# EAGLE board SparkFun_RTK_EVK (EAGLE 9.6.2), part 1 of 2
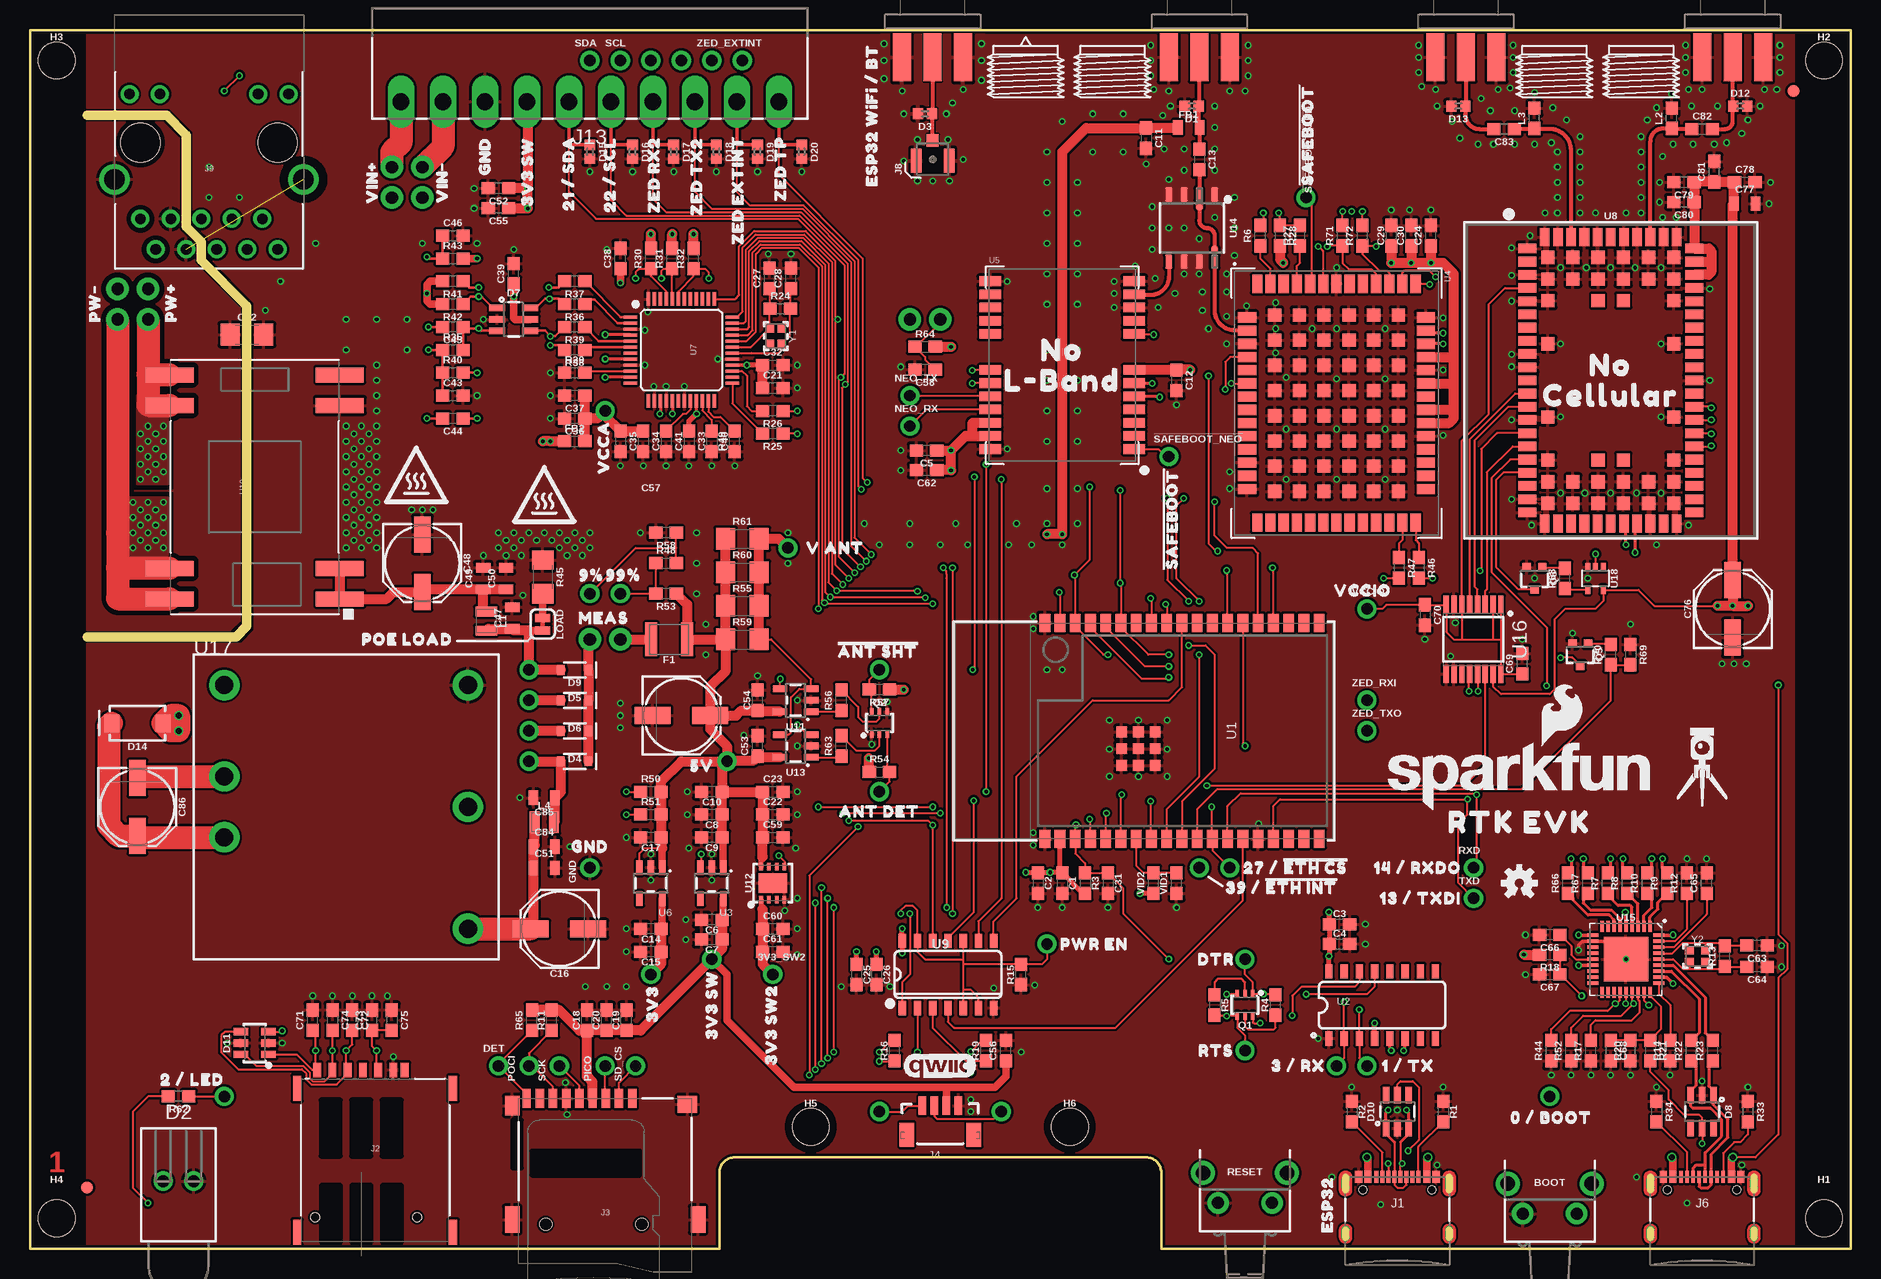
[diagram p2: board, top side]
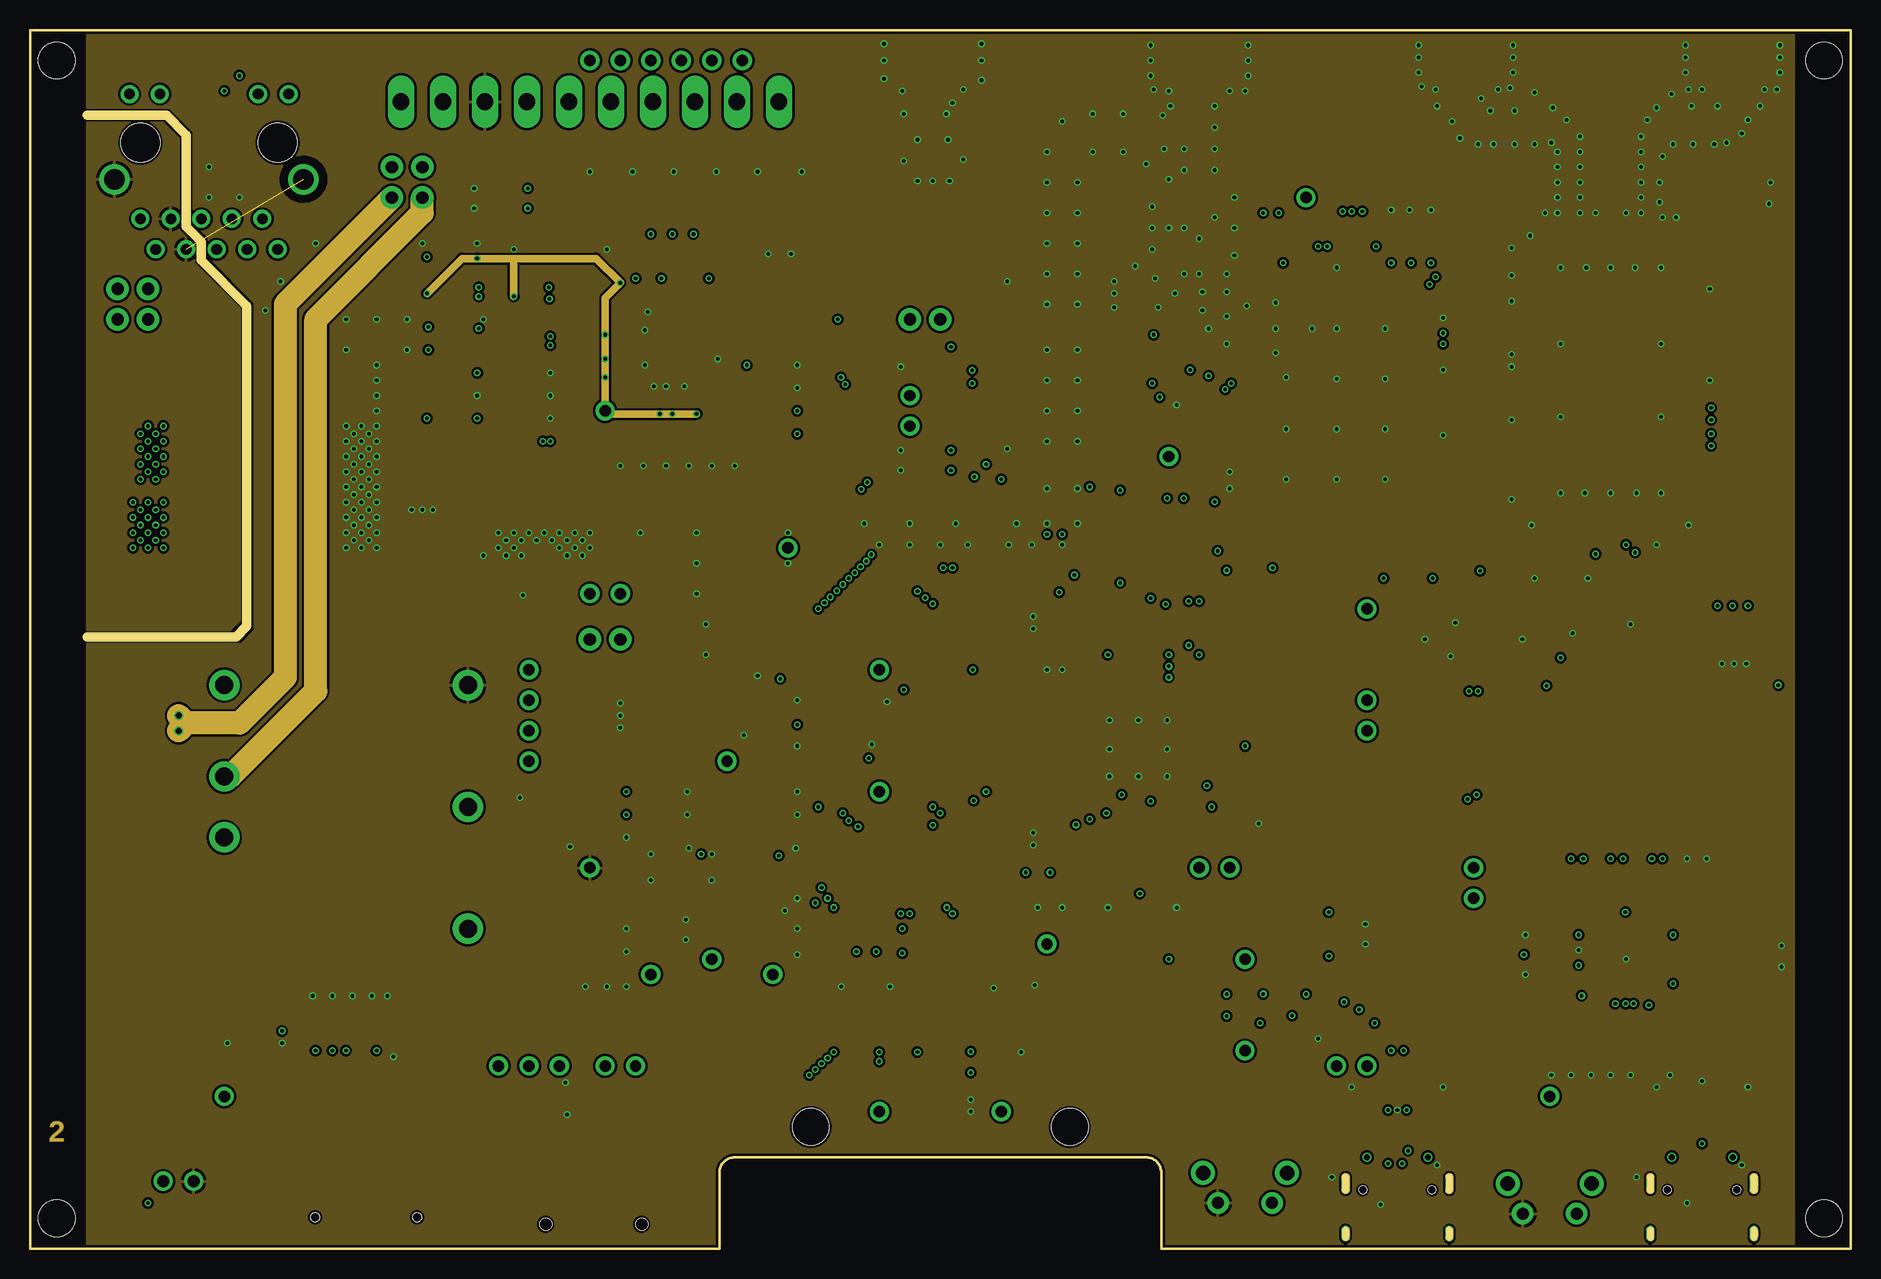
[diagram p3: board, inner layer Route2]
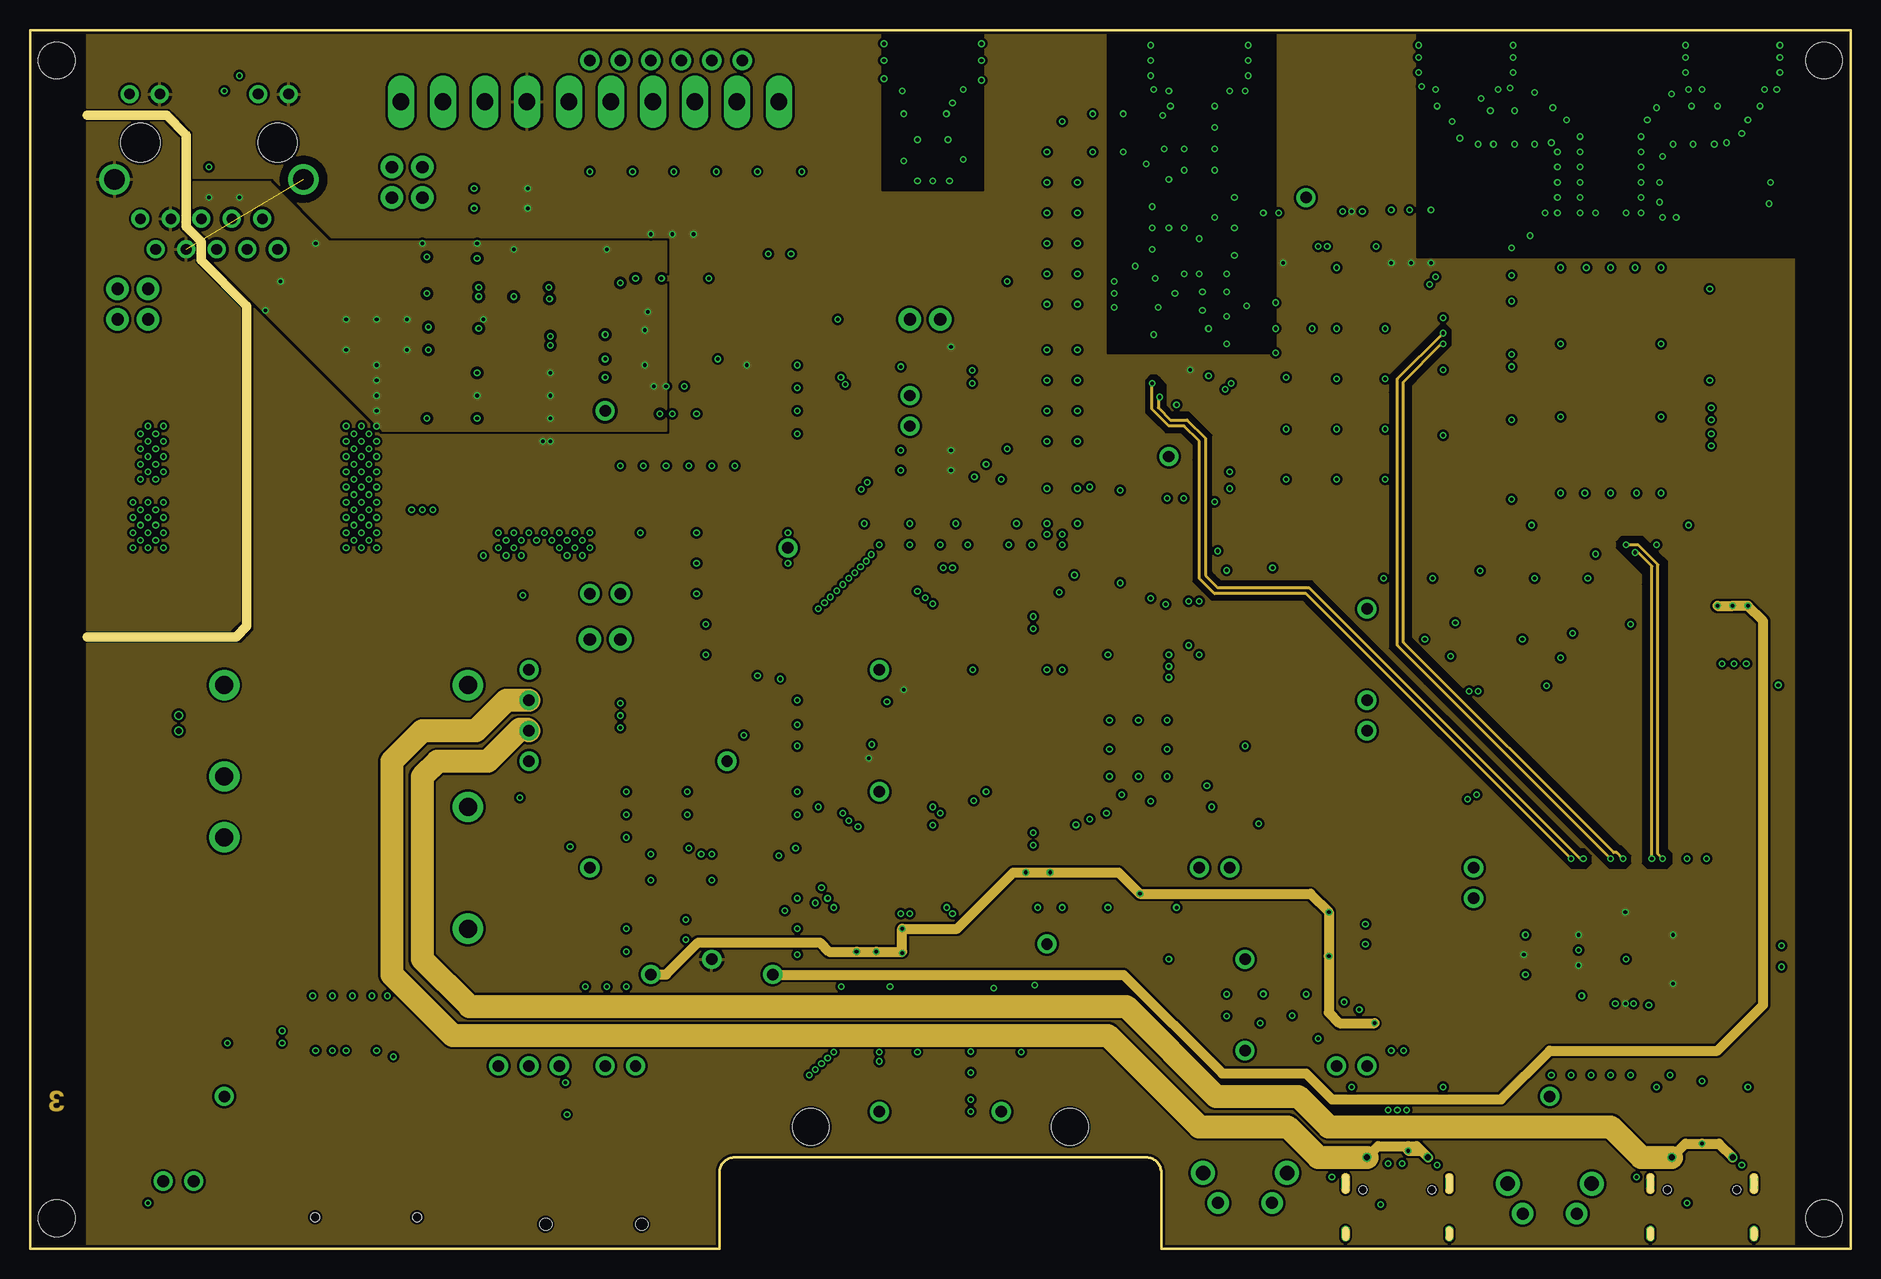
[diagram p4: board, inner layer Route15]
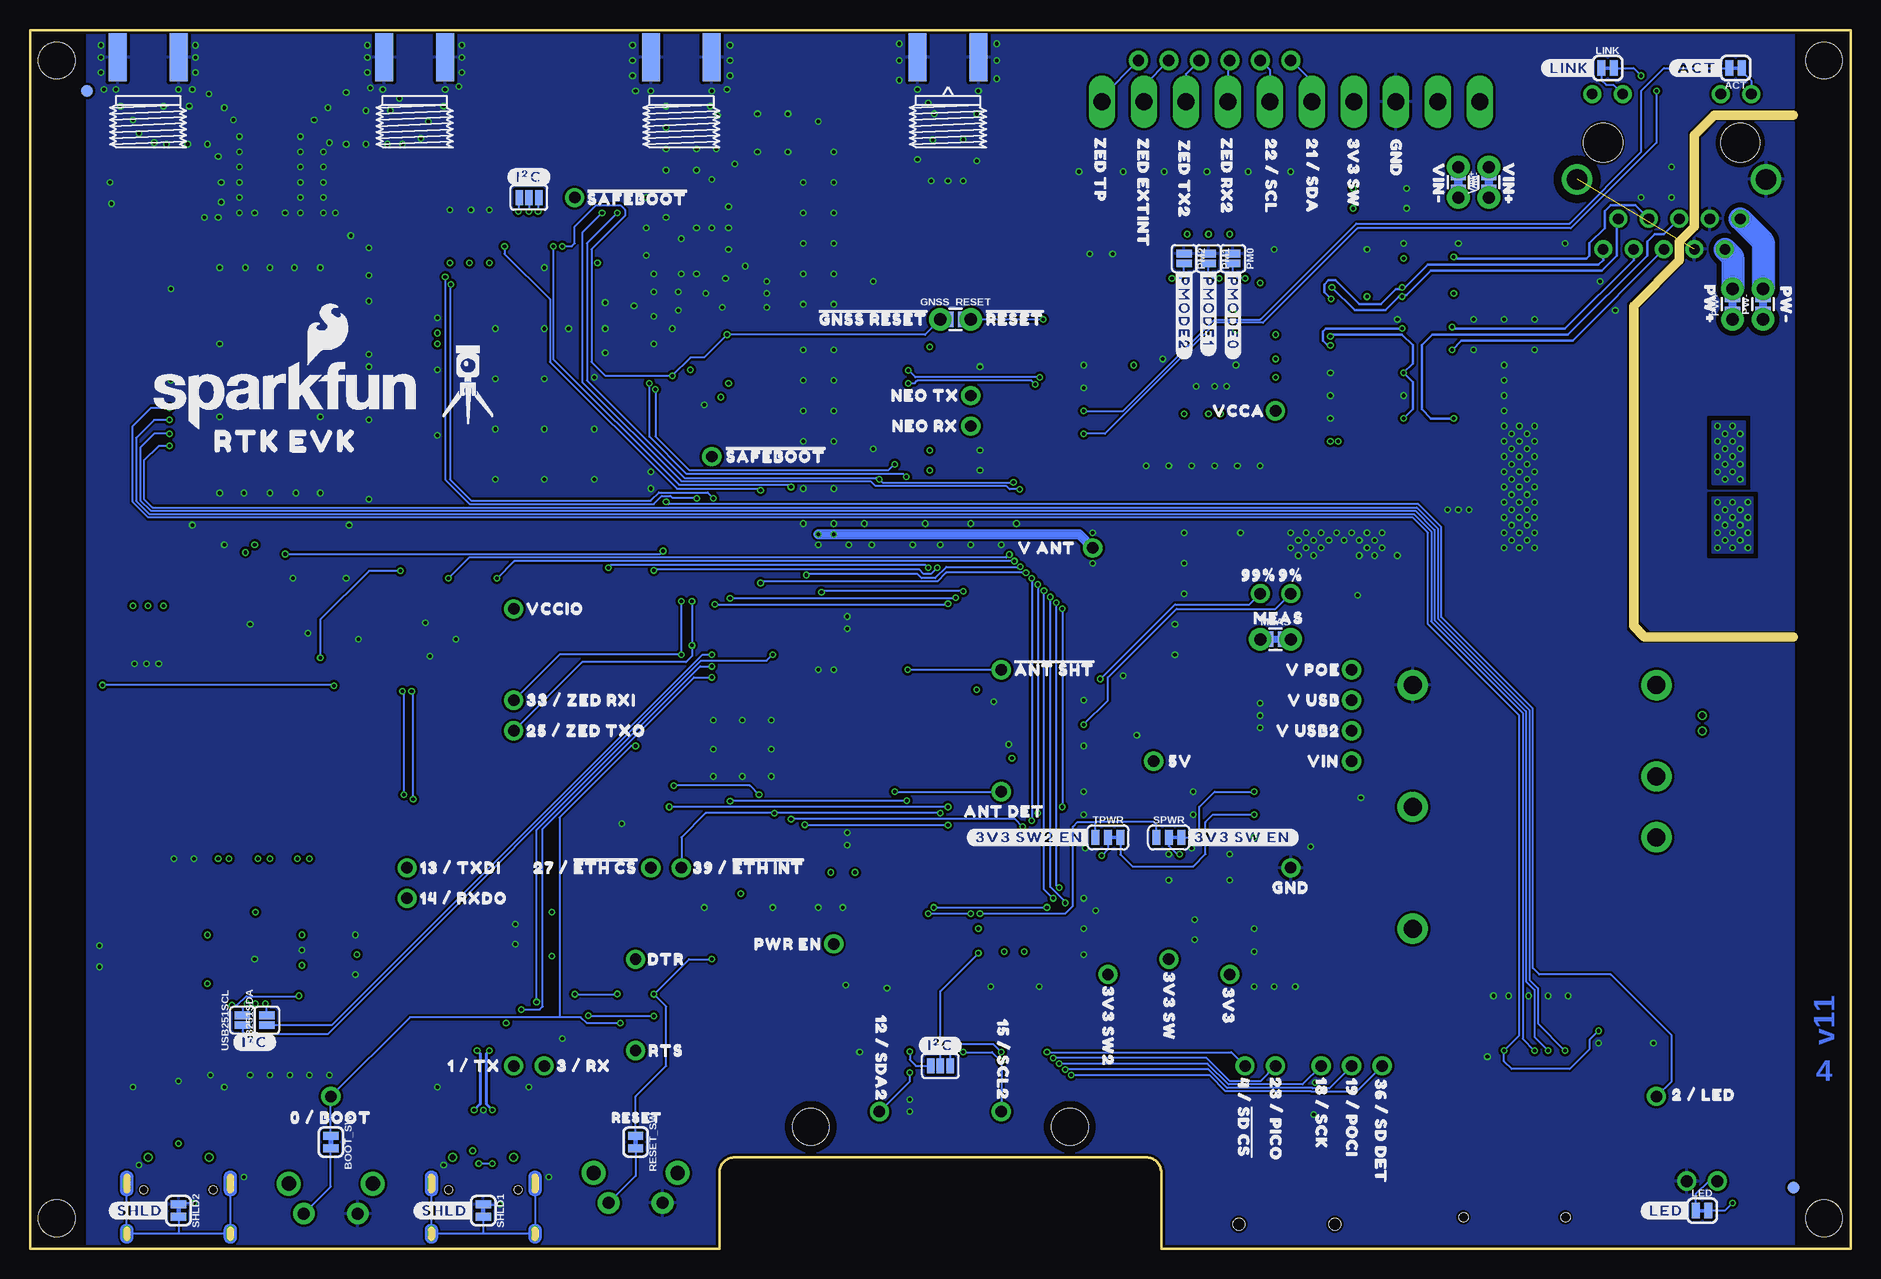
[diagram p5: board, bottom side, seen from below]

Size 151.77 x 101.6 mm. Coordinates in mm from the lower left corner, seen from the top.
Outline: 0,0 57.47,0 57.47,6.35 arc-90 58.74,7.62 93.03,7.62 arc-90 94.3,6.35 94.3,0 151.77,0 151.77,101.6 0,101.6 0,0
Copper layers (1*2*15*16): Top 0.035559375mm / dielectric 0.47751875mm / Route2 0.035559375mm / dielectric 0.47751875mm / Route15 0.035559375mm / dielectric 0.47751875mm / Bottom 0.035559375mm
Design rules "SparkFun-4-Layer-Minimum-JLCPCB": minimum track width 5mil, minimum drill 0.2mm, track to track 5mil, track to pad 5mil, pad to pad 5mil, via to via 5mil, smd to smd 5mil, copper to edge 7mil, drill to drill 7mil, minimum pad ring 5mil, minimum via ring 5mil, stop-mask expansion 2.5mil, vias tented up to drill 25mil, thermal gap 10mil
Net classes: 2 3.3V: width 0.508 mm; 3 RF_IN: width 0.35 mm, clearance 0.46 mm; 4 USB: width 0.203 mm, clearance 0.127 mm; 7 V_ZED: width 0.2 mm, clearance 0.2 mm; 8 V_RF: width 0.2 mm; 11 ZED_DIG: width 0.1 mm, clearance 0.1 mm
tKeepout: area 0,6.3 to 4.8,95.2; area 147,6.3 to 151.8,95.2
tRestrict: 1 lines
Milling: 9 lines

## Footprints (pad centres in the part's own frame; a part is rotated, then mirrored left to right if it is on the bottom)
1X01_NO_SILK = drill 0.95 pad 1.6: 1 0,0
SMT-JUMPER_2_NC_TRACE_SILK = smd 0.66 x 1.27: 1 -0.521,0; 2 0.521,0
TACTILE_SWITCH_PTH_RA_8-020 = drill 1 pad 1.8: 1 -2.25,0; 2 2.25,0 | drill 1.2 pad 2: M1 -3.5,2.5; M2 3.5,2.5
SMT-JUMPER_2_SOIC-PAD_NO-PASTE = smd 0.55 x 0.55: 1 1.75,0
0603 = smd 1.1 x 1: 1 -0.85,0; 2 0.85,0
PANASONIC_D = smd 3 x 1.4: + 2.4,0; - -2.4,0
1206 = smd 1.6 x 1.8: 1 -1.4,0; 2 1.4,0
0805 = smd 0.8 x 1.2: 1 -0.9,0; 2 0.9,0
0402 = smd 0.85 x 0.9: 1 -0.58,0; 2 0.58,0
CBI-RIGHT-ANGLE-PTH = drill 1 pad 1.6: A -1.27,5; C 1.27,5
SOD-323 = smd 0.63 x 0.83: A 1.15,0; C -1.15,0
SOT-23-6 = smd 0.55 x 1.35: 1 -0.95,-1.375; 2 0,-1.375; 3 0.95,-1.375; 4 0.95,1.375; 5 0,1.375; 6 -0.95,1.375
SOT23-6L = smd 0.6 x 1.2: 1 -0.95,-1.15; 2 0,-1.15; 3 0.95,-1.15; 4 0.95,1.15; 5 0,1.15; 6 -0.95,1.15
SMA-DIODE = smd 1.27 x 1.47: A -2.15,0; C 2.15,0
RP-SMA-EDGE = smd 1.5 x 4: GND@0 -2.54,0; GND@1 2.54,0; SIG 0,0 | smd 1.5 x 4 bottom: GND@2 -2.54,0; GND@3 2.54,0
1210 = smd 1 x 2.8: 1 -1.5,0; 2 1.5,0
FIDUCIAL-1X2 = smd 1 x 1: 1 0,0
COMBO-JUMPER_2_NO = smd 0.635 x 1.27: 1 -0.508,0; 2 0.508,0 | drill 1.016 pad 1.88: 3 -1.27,0; 4 1.27,0
SMA-EDGE = smd 1.5 x 4: GND@0 -2.54,0; GND@1 2.54,0; SIG 0,0 | smd 1.5 x 4 bottom: GND@2 -2.54,0; GND@3 2.54,0
STAND-OFF-TIGHT = hole 3.048: 0,0
SMT-JUMPER_3_NO_SILK = smd 0.635 x 1.27: 1 -0.813,0; 2 0,0; 3 0.813,0
USB-C-16P_4LAYER-PADS = smd 0.3 x 1: A5 -1.25,-0.34; A6 -0.25,-0.34; A7 0.25,-0.34; A8 1.25,-0.34; B5 1.75,-0.34; B6 0.75,-0.34; B7 -0.75,-0.34; B8 -1.75,-0.34 | smd 0.6 x 1: GND -3.225,-0.34; GND2 3.225,-0.34; VBUS1 -2.45,-0.34; VBUS2 2.45,-0.34 | drill 0.4 pad 0.6 long: SHLD1 -4.318,-0.915; SHLD2 4.318,-0.915; SHLD3 -4.318,-5.095; SHLD4 4.318,-5.095 | hole 0.65: -2.89,-1.445; 2.89,-1.445
NANO_SIM_PP = smd 0.7 x 2.1: A1 6.495,6; A2 -6.495,6; A3 -6.495,-6; A4 6.495,-6 | smd 0.65 x 1.23: C1 0.255,7.535; C2 -2.285,7.535; C3 -4.825,7.535; C5 1.525,7.535; C6 -1.015,7.535; C7 -3.555,7.535; CD 2.475,7.535 | hole 0.75: 3.505,-4.75; -4.995,-4.75
MICROSD-EXTERNALPIN = smd 0.7 x 1.6: 1 2.25,10.5; 2 1.15,10.5; 3 0.05,10.5; 4 -1.05,10.5; 5 -2.15,10.5; 6 -3.25,10.5; 7 -4.35,10.5; 8 -5.45,10.5; 9 -6.55,10.5 | smd 1.2 x 1.6: 10 -7.75,9.9 | smd 1.2 x 2.2: 11 -7.75,0.4; 12 7.75,0.4 | smd 1.6 x 1.4: 13 6.85,10 | hole 1: 3.05,0; -4.95,0
JST04_1MM_VERT = smd 0.6 x 1.55: 1 -1.5,0.775; 2 -0.5,0.775; 3 0.5,0.775; 4 1.5,0.775 | smd 1.2 x 2: NC1 -2.8,3.2; NC2 2.8,3.2
U.FL_REDUCED_FOOTPRINT = smd 2 x 0.85: 1 -0.1,1.375; 2 -0.1,-1.375 | smd 1.05 x 1: FEED 1.575,0
MAGJACK-SYM_LED = drill 0.9 pad 1.5: 1 -5.715,8.89; 2 -4.445,6.35; 3 -3.175,8.89; 4 -1.905,6.35; 5 -0.635,8.89; 6 0.635,6.35; 7 1.905,8.89; 8 3.175,6.35; 9 4.445,8.89; 10 5.715,6.35; 11 -6.63,-4.06; 12 -4.09,-4.06; 13 4.09,-4.06; 14 6.63,-4.06 | drill 1.7 pad 2.4: S1 -7.875,3.05; S2 7.875,3.05 | hole 3.25: -5.715,0; 5.715,0
1X10_SCREW_TERMINAL_3.5MM = drill 1.4 pad 2.2 long: 1 -15.75,2.8; 2 -12.25,2.8; 3 -8.75,2.8; 4 -5.25,2.8; 5 -1.75,2.8; 6 1.75,2.8; 7 5.25,2.8; 8 8.75,2.8; 9 12.25,2.8; 10 15.75,2.8
0805-WIDE = smd 0.8 x 1.8: 1 -0.8,0; 2 0.8,0
0603_NO-CREAM = smd 1.1 x 1: 1 -0.85,0; 2 0.85,0
COMBO-JUMPER_2_NC_TRACE = smd 0.635 x 1.27: 1 -0.508,0; 2 0.508,0 | drill 1.016 pad 1.88: 3 -1.27,0; 4 1.27,0
SMT-JUMPER_2_NO_SILK = smd 0.635 x 1.27: 1 -0.406,0; 2 0.406,0
SC70-6 = smd 0.3 x 0.66: 1 -0.65,-0.92; 2 0,-0.92; 3 0.65,-0.92; 4 0.65,0.92; 5 0,0.92; 6 -0.65,0.92
SOT323 = smd 0.7 x 0.7: 1 -0.65,-0.925; 2 0.65,-0.925; 3 0,0.925
SMT-JUMPER_3_1-NC_TRACE_SILK = smd 0.66 x 1.27: 1 -1.041,0; 2 0,0; 3 1.041,0
ESP32-WROVER-E/IE = smd 0.9 x 1.5: 1 7.8,9; 2 6.53,9; 3 5.26,9; 4 3.99,9; 5 2.72,9; 6 1.45,9; 7 0.18,9; 8 -1.09,9; 9 -2.36,9; 10 -3.63,9; 11 -4.9,9; 12 -6.17,9; 13 -7.44,9; 14 -8.71,9; 15 -9.98,9; 16 -11.25,9; 17 -12.52,9; 18 -13.79,9; 19 -15.06,9; 20 -15.06,-9; 21 -13.79,-9; 22 -12.52,-9; 23 -11.25,-9; 24 -9.98,-9; 25 -8.71,-9; 26 -7.44,-9; 27 -6.17,-9; 28 -4.9,-9; 29 -3.63,-9; 30 -2.36,-9; 31 -1.09,-9; 32 0.18,-9; 33 1.45,-9; 34 2.72,-9; 35 3.99,-9; 36 5.26,-9; 37 6.53,-9; 38 7.8,-9 | smd 0.9 x 0.9: GND 0,1.5; GNDT1 -1.4,2.9; GNDT2 -1.4,1.5; GNDT3 -1.4,0.1; GNDT4 0,0.1; GNDT5 1.4,0.1; GNDT6 1.4,1.5; GNDT7 1.4,2.9; GNDT8 0,2.9
SO016 = smd 0.6 x 1.2: 1 -4.445,-2.8; 2 -3.175,-2.8; 3 -1.905,-2.8; 4 -0.635,-2.8; 5 0.635,-2.8; 6 1.905,-2.8; 7 3.175,-2.8; 8 4.445,-2.8; 9 4.445,2.8; 10 3.175,2.8; 11 1.905,2.8; 12 0.635,2.8; 13 -0.635,2.8; 14 -1.905,2.8; 15 -3.175,2.8; 16 -4.445,2.8
SOT23-5 = smd 0.55 x 1.2: 1 -0.95,-1.3; 2 0,-1.3; 3 0.95,-1.3; 4 0.95,1.3; 5 -0.95,1.3
ZED-F9P = smd 0.85 x 1.52: 1 -7.15,-7.45; 2 -6.05,-7.45; 3 -4.95,-7.45; 4 -3.85,-7.45; 5 -2.75,-7.45; 6 -1.65,-7.45; 7 -0.55,-7.45; 8 0.55,-7.45; 9 1.65,-7.45; 10 2.75,-7.45; 11 3.85,-7.45; 12 4.95,-7.45; 13 6.05,-7.45; 14 7.15,-7.45; 28 7.15,7.45; 29 6.05,7.45; 30 4.95,7.45; 31 3.85,7.45; 32 2.75,7.45; 33 1.65,7.45; 34 0.55,7.45; 35 -0.55,7.45; 36 -1.65,7.45; 37 -2.75,7.45; 38 -3.85,7.45; 39 -4.95,7.45; 40 -6.05,7.45; 41 -7.15,7.45 | smd 1.52 x 0.85: 15 9.95,-6.6; 16 9.95,-5.5; 17 9.95,-4.4; 18 9.95,-3.3; 19 9.95,-2.2; 20 9.95,-1.1; 21 9.95,0; 22 9.95,1.1; 23 9.95,2.2; 24 9.95,3.3; 25 9.95,4.4; 26 9.95,5.5; 27 9.95,6.6; 42 -9.95,6.6; 43 -9.95,5.5; 44 -9.95,4.4; 45 -9.95,3.3; 46 -9.95,2.2; 47 -9.95,1.1; 48 -9.95,0; 49 -9.95,-1.1; 50 -9.95,-2.2; 51 -9.95,-3.3; 52 -9.95,-4.4; 53 -9.95,-5.5; 54 -9.95,-6.6 | smd 1.1 x 1.1: 55 -1.05,-1.05; 56 -3.15,-1.05; 57 -5.25,-1.05; 58 -7.35,-1.05; 59 -1.05,-3.1; 60 -3.15,-3.1; 61 -5.25,-3.1; 62 -7.35,-3.1; 63 -1.05,-5.15; 64 -3.15,-5.15; 65 -5.25,-5.15; 66 -7.35,-5.15; 67 -1.05,5.15; 68 -3.15,5.15; 69 -5.25,5.15; 70 -7.35,5.15; 71 -1.05,3.1; 72 -3.15,3.1; 73 -5.25,3.1; 74 -7.35,3.1; 75 -1.05,1.05; 76 -3.15,1.05; 77 -5.25,1.05; 78 -7.35,1.05; 79 1.05,1.05; 80 3.15,1.05; 81 5.25,1.05; 82 7.35,1.05; 83 1.05,3.1; 84 3.15,3.1; 85 5.25,3.1; 86 7.35,3.1; 87 1.05,5.15; 88 3.15,5.15; 89 5.25,5.15; 90 7.35,5.15; 91 1.05,-5.15; 92 3.15,-5.15; 93 5.25,-5.15; 94 7.35,-5.15; 95 1.05,-3.1; 96 3.15,-3.1; 97 5.25,-3.1; 98 7.35,-3.1; 99 1.05,-1.05; 100 3.15,-1.05; 101 5.25,-1.05; 102 7.35,-1.05
NEO-M9N/M8T/M8U/D9S = smd 1.8 x 0.8: 1 6,-7; 2 6,-5.9; 3 6,-4.8; 4 6,-3.7; 5 6,-2.6; 6 6,-1.5; 7 6,-0.4; 8 6,2.6; 9 6,3.7; 10 6,4.8; 11 6,5.9; 12 6,7; 13 -6,7; 14 -6,5.9; 15 -6,4.8; 16 -6,3.7; 17 -6,2.6; 18 -6,-0.4; 19 -6,-1.5; 20 -6,-2.6; 21 -6,-3.7; 22 -6,-4.8; 23 -6,-5.9; 24 -6,-7
LQFP-48 = smd 0.254 x 1.143: 1 -2.75,-4.25; 2 -2.25,-4.25; 3 -1.75,-4.25; 4 -1.25,-4.25; 5 -0.75,-4.25; 6 -0.25,-4.25; 7 0.25,-4.25; 8 0.75,-4.25; 9 1.25,-4.25; 10 1.75,-4.25; 11 2.25,-4.25; 12 2.75,-4.25; 25 2.75,4.25; 26 2.25,4.25; 27 1.75,4.25; 28 1.25,4.25; 29 0.75,4.25; 30 0.25,4.25; 31 -0.25,4.25; 32 -0.75,4.25; 33 -1.25,4.25; 34 -1.75,4.25; 35 -2.25,4.25; 36 -2.75,4.25 | smd 1.143 x 0.254: 13 4.25,-2.75; 14 4.25,-2.25; 15 4.25,-1.75; 16 4.25,-1.25; 17 4.25,-0.75; 18 4.25,-0.25; 19 4.25,0.25; 20 4.25,0.75; 21 4.25,1.25; 22 4.25,1.75; 23 4.25,2.25; 24 4.25,2.75; 37 -4.25,2.75; 38 -4.25,2.25; 39 -4.25,1.75; 40 -4.25,1.25; 41 -4.25,0.75; 42 -4.25,0.25; 43 -4.25,-0.25; 44 -4.25,-0.75; 45 -4.25,-1.25; 46 -4.25,-1.75; 47 -4.25,-2.25; 48 -4.25,-2.75
LARA-LGA = smd 0.8 x 1.5: 1 -11,-6.95; 2 -9.9,-6.95; 3 -8.8,-6.95; 4 -7.7,-6.95; 5 -6.6,-6.95; 6 -5.5,-6.95; 7 -4.4,-6.95; 8 -3.3,-6.95; 9 -2.2,-6.95; 10 -1.1,-6.95; 11 0,-6.95; 12 1.1,-6.95; 13 2.2,-6.95; 14 3.3,-6.95; 15 4.4,-6.95; 16 5.5,-6.95; 17 6.6,-6.95; 18 7.7,-6.95; 19 8.8,-6.95; 20 9.9,-6.95; 21 11,-6.95; 33 11,6.95; 34 9.9,6.95; 35 8.8,6.95; 36 7.7,6.95; 37 6.6,6.95; 38 5.5,6.95; 39 4.4,6.95; 40 3.3,6.95; 41 2.2,6.95; 42 1.1,6.95; 43 0,6.95; 44 -1.1,6.95; 45 -2.2,6.95; 46 -3.3,6.95; 47 -4.4,6.95; 48 -5.5,6.95; 49 -6.6,6.95; 50 -7.7,6.95; 51 -8.8,6.95; 52 -9.9,6.95; 53 -11,6.95 | smd 1.5 x 0.8: 22 11.95,-5.5; 23 11.95,-4.4; 24 11.95,-3.3; 25 11.95,-2.2; 26 11.95,-1.1; 27 11.95,0; 28 11.95,1.1; 29 11.95,2.2; 30 11.95,3.3; 31 11.95,4.4; 32 11.95,5.5; 54 -11.95,5.5; 55 -11.95,4.4; 56 -11.95,3.3; 57 -11.95,2.2; 58 -11.95,1.1; 59 -11.95,0; 60 -11.95,-1.1; 61 -11.95,-2.2; 62 -11.95,-3.3; 63 -11.95,-4.4; 64 -11.95,-5.5 | smd 1.1 x 1.1: 65 -10.25,-5.25; 66 -10.25,-3.15; 67 -10.25,-1.05; 68 -10.25,1.05; 69 -10.25,3.15; 70 -10.25,5.25; 71 -8.45,-5.25; 72 -8.45,-3.15; 73 -8.45,-1.05; 74 -8.45,1.05; 75 -8.45,3.15; 76 -8.45,5.25; 77 -6.65,-5.25; 78 -6.65,5.25; 79 -3.05,-5.25; 80 -3.05,5.25; 81 3.05,-5.25; 82 3.05,5.25; 83 6.65,-5.25; 84 6.65,5.25; 85 8.45,-5.25; 86 8.45,-3.15; 87 8.45,-1.05; 88 8.45,1.05; 89 8.45,3.15; 90 8.45,5.25; 91 10.25,-5.25; 92 10.25,-3.15; 93 10.25,-1.05; 94 10.25,1.05; 95 10.25,3.15; 96 10.25,5.25; 97 -6.65,-1.05; 98 -6.65,1.05; 99 6.65,-1.05; 100 6.65,1.05
SO14 = smd 0.6 x 1.2: 1 -3.175,-2.8; 2 -1.905,-2.8; 3 -0.635,-2.8; 4 0.635,-2.8; 5 1.905,-2.8; 6 3.175,-2.8; 7 4.445,-2.8; 8 4.445,2.8; 9 3.175,2.8; 10 1.905,2.8; 11 0.635,2.8; 12 -0.635,2.8; 13 -1.905,2.8; 14 -3.175,2.8
DP990X = smd 1.25 x 4: 1 -9.33,-7.1; 2 -6.79,-7.1; 3 6.79,-7.1; 4 9.33,-7.1; 5 9.33,7.1; 6 6.79,7.1; 7 -6.79,7.1; 8 -9.33,7.1
UDFN-8 = smd 0.3 x 0.65: 1 -0.975,-1.375; 2 -0.325,-1.375; 3 0.325,-1.375; 4 0.975,-1.375; 5 0.975,1.375; 6 0.325,1.375; 7 -0.325,1.375; 8 -0.975,1.375 | smd 2.35 x 1.6: EP 0,0
XX21 = smd 0.6 x 1.2: 1 -1.905,-2.8; 2 -0.635,-2.8; 3 0.635,-2.8; 4 1.905,-2.8; 5 1.905,2.8; 6 0.635,2.8; 7 -0.635,2.8; 8 -1.905,2.8
QFN-36 = smd 0.9 x 0.28: 1 -2.75,2; 2 -2.75,1.5; 3 -2.75,1; 4 -2.75,0.5; 5 -2.75,0; 6 -2.75,-0.5; 7 -2.75,-1; 8 -2.75,-1.5; 9 -2.75,-2; 19 2.75,-2; 20 2.75,-1.5; 21 2.75,-1; 22 2.75,-0.5; 23 2.75,0; 24 2.75,0.5; 25 2.75,1; 26 2.75,1.5; 27 2.75,2 | smd 0.28 x 0.9: 10 -2,-2.75; 11 -1.5,-2.75; 12 -1,-2.75; 13 -0.5,-2.75; 14 0,-2.75; 15 0.5,-2.75; 16 1,-2.75; 17 1.5,-2.75; 18 2,-2.75; 28 2,2.75; 29 1.5,2.75; 30 1,2.75; 31 0.5,2.75; 32 0,2.75; 33 -0.5,2.75; 34 -1,2.75; 35 -1.5,2.75; 36 -2,2.75 | smd 3.7 x 3.7: EP 0,0
SOP65P640X120-16N = smd 1.5 x 0.45: 1 -2.9,2.275; 2 -2.9,1.625; 3 -2.9,0.975; 4 -2.9,0.325; 5 -2.9,-0.325; 6 -2.9,-0.975; 7 -2.9,-1.625; 8 -2.9,-2.275; 9 2.9,-2.275; 10 2.9,-1.625; 11 2.9,-0.975; 12 2.9,-0.325; 13 2.9,0.325; 14 2.9,0.975; 15 2.9,1.625; 16 2.9,2.275
URB_YMD-15WR3 = drill 1.499 pad 2.54: 1 -10.16,10.16; 2 -10.16,2.54; 3 -10.16,-2.54; 4 10.16,-10.16; 5 10.16,0; 6 10.16,10.16
SOT353 = smd 0.42 x 0.7: 1 -0.65,-0.95; 2 0,-0.95; 3 0.65,-0.95; 4 0.65,0.95; 5 -0.65,0.95
CRYSTAL-SMD-2.0X1.6MM = smd 0.75 x 0.7: 1 -0.675,-0.5; 2 0.675,-0.5; 3 0.675,0.5; 4 -0.675,0.5

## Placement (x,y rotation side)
3V3  TEST-POINTPOGO_PTH  [1X01_NO_SILK]  51.75,22.86 270 top
3V3_SW  TEST-POINTPOGO_PTH  [1X01_NO_SILK]  56.83,24.13 270 top
3V3_SW2  TEST-POINTPOGO_PTH  [1X01_NO_SILK]  61.91,22.86 0 top
5V  TEST-POINTPOGO_PTH  [1X01_NO_SILK]  58.1,40.64 270 top
9%  TEST-POINTPOGO_PTH  [1X01_NO_SILK]  46.67,54.61 0 top
99%  TEST-POINTPOGO_PTH  [1X01_NO_SILK]  49.21,54.61 0 top
!SAFEBOOT_NEO!  TEST-POINTPOGO_PTH  [1X01_NO_SILK]  94.93,66.04 0 top
!SAFEBOOT_ZED!  TEST-POINTPOGO_PTH  [1X01_NO_SILK]  106.36,87.63 0 top
ACT  JUMPER-SMT_2_NC_TRACE_SILK  [SMT-JUMPER_2_NC_TRACE_SILK]  9.59,98.42 180 bottom
ANT_DET  TEST-POINTPOGO_PTH  [1X01_NO_SILK]  70.8,38.1 0 top
ANT_SHT  TEST-POINTPOGO_PTH  [1X01_NO_SILK]  70.8,48.26 0 top
BOOT  MOMENTARY-SWITCH-SPST-PTH-RIGHT-ANGLE-8-020  [TACTILE_SWITCH_PTH_RA_8-020]  126.68,2.92 0 top
BOOT_SW  JUMPER-SMT_2_NC_TRACE_SILK  [SMT-JUMPER_2_NC_TRACE_SILK]  126.68,8.89 270 bottom
BYPASS1  NO PASTE  [SMT-JUMPER_2_SOIC-PAD_NO-PASTE]  97.47,85.09 90 top
BYPASS2  NO PASTE  [SMT-JUMPER_2_SOIC-PAD_NO-PASTE]  98.74,85.09 270 top
C1  2.2uF  [0603]  86.04,30.48 270 top
C2  0.1uF  [0603]  84.01,30.48 270 top
C3  2.2uF  [0603]  109.16,27.05 0 top
C4  10nF  [0603]  109.16,25.4 0 top
C5  2.2uF  [0603]  74.74,66.55 180 top
C6  2.2uF  [0603]  56.83,27.43 180 top
C7  0.1uF  [0603]  56.83,25.78 180 top
C8  2.2uF  [0603]  56.83,36.2 180 top
C9  2.2uF  [0603]  56.83,34.29 180 top
C10  2.2uF  [0603]  56.83,38.1 180 top
C11  47pF  [0603]  93.03,92.58 270 top
C12  1.0uF  [0603]  95.57,72.39 270 top
C13  47pF  [0603]  97.47,90.81 270 top
C14  2.2uF  [0603]  51.75,26.67 180 top
C15  0.1uF  [0603]  51.75,24.77 180 top
C16  100uF  [PANASONIC_D]  44.13,26.67 180 top
C17  0.1uF  [0603]  51.75,34.29 180 top
C18  2.2uF  [0603]  46.42,19.05 90 top
C19  0.1uF  [0603]  49.72,19.05 90 top
C20  10uF  [0603]  48.07,19.05 90 top
C21  0.1uF  [0603]  61.91,71.75 0 top
C22  2.2uF  [0603]  61.91,36.2 0 top
C23  2.2uF  [0603]  61.91,38.1 0 top
C24  1.0uF  [0603]  116.78,84.45 90 top
C25  2.2uF  [0603]  68.9,22.86 270 top
C26  2.2uF  [0603]  70.55,22.86 270 top
C27  10pF  [0603]  61.66,80.9 90 top
C28  10pF  [0603]  63.44,80.9 90 top
C29  2.2uF  [0603]  113.47,84.45 90 top
C30  0.1uF  [0603]  115.13,84.45 90 top
C31  0.1uF  [0603]  89.85,30.48 270 top
C32  10uF  [0603]  61.91,73.66 0 top
C33  0.1uF  [0603]  54.93,67.31 270 top
C34  0.1uF  [0603]  51.12,67.31 270 top
C35  0.1uF  [0603]  49.21,67.31 270 top
C36  0.1uF  [0603]  45.4,69.22 180 top
C37  0.1uF  [0603]  45.4,71.12 180 top
C38  0.1uF  [0603]  49.21,82.55 90 top
C39  10uF  [0603]  40.32,81.28 90 top
C40  10nF  [0603]  56.83,67.31 270 top
C41  4.7uF  [0603]  53.02,67.31 270 top
C42  1nF  [1206]  18.08,76.2 0 top
C43  10nF  [0603]  35.24,71.12 0 top
C44  6.8nF  [0603]  35.24,69.22 180 top
C45  6.8nF  [0603]  35.24,76.83 180 top
C46  22nF  [0603]  35.24,84.45 0 top
C47  10uF  [0805]  40.2,52.58 90 top
C48  100uF  [PANASONIC_D]  32.7,57.15 270 top
C49  10uF  [0805]  37.78,55.88 90 top
C50  10uF  [0805]  39.69,55.88 90 top
C51  10uF  [0805]  42.86,31.75 0 top
C52  0.1uF  [0603]  39.05,88.39 180 top
C53  0.1uF  [0603]  60.64,41.91 90 top
C54  0.1uF  [0603]  60.64,45.72 90 top
C55  10uF  [0603]  39.05,86.74 180 top
C56  2.2uF  [0603]  81.34,16.51 90 top
C57  100uF  [PANASONIC_D]  54.29,44.45 0 top
C58  0.1uF  [0603]  74.61,73.28 180 top
C59  2.2uF  [0603]  61.91,34.29 0 top
C60  2.2uF  [0603]  61.91,26.67 0 top
C61  0.1uF  [0603]  61.91,24.77 0 top
C62  0.1uF  [0603]  74.74,64.9 180 top
C63  18pF  [0603]  143.95,25.27 180 top
C64  18pF  [0603]  143.95,23.5 180 top
C65  0.1uF  [0603]  139.76,30.48 90 top
C66  0.1uF  [0603]  126.68,26.16 180 top
C67  0.1uF  [0603]  126.68,22.86 180 top
C68  0.1uF  [0603]  131.76,16.51 270 top
C69  0.1uF  [0603]  124.4,48.77 90 top
C70  0.1uF  [0603]  116.27,52.83 270 top
C71  47pF  [0603]  23.56,19.05 90 top
C72  47pF  [0603]  26.86,19.05 270 top
C73  47pF  [0603]  28.51,19.05 90 top
C74  47pF  [0603]  25.21,19.05 270 top
C75  0.1uF  [0603]  30.16,19.05 270 top
C76  100uF  [PANASONIC_D]  141.92,53.34 90 top
C77  10uF  [0805]  142.94,87.12 0 top
C78  0.1uF  [0603]  142.94,88.9 0 top
C79  15pF  [0603]  137.86,88.9 180 top
C80  8.2pF  [0603]  137.86,87.25 180 top
C81  68pF  [0603]  140.4,89.79 90 top
C82  33pF  [0603]  139.38,93.34 0 top
C83  33pF  [0603]  122.87,93.34 180 top
C84  10uF  [0805]  42.86,33.53 0 top
C85  10uF  [0805]  42.86,37.59 180 top
C86  47UF  [PANASONIC_D]  8.95,36.83 270 top
D1  PESD0402-0402  [0402]  96.84,95.25 180 top
D2  LED-RIGHT-ANGLE-PTH-GREEN  [CBI-RIGHT-ANGLE-PTH]  12.38,0.64 0 top
D3  PESD0402  [0402]  74.61,94.61 180 top
D4  3A/10V/280mV  [SOD-323]  45.4,40.64 180 top
D5  3A/10V/280mV  [SOD-323]  45.4,45.72 180 top
D6  3A/10V/280mV  [SOD-323]  45.4,43.18 180 top
D7  ESD Diode  [SOT-23-6]  40.32,77.47 270 top
D8  ESD Diode  [SOT-23-6]  139.38,11.43 180 top
D9  3A/10V/280mV  [SOD-323]  45.4,48.26 180 top
D10  ESD Diode  [SOT-23-6]  113.98,11.43 0 top
D11  TVS_DIODE  [SOT23-6L]  18.73,17.14 90 top
D12  PESD0402-0402  [0402]  142.56,95.25 0 top
D13  PESD0402-0402  [0402]  119.06,95.25 180 top
D14  3A/40V  [SMA-DIODE]  8.95,43.81 180 top
D15  PESD0402-0402  [0402]  46.67,91.44 270 top
D16  PESD0402-0402  [0402]  50.23,91.44 270 top
D17  PESD0402-0402  [0402]  53.66,91.44 270 top
D18  PESD0402-0402  [0402]  57.21,91.44 270 top
D19  PESD0402-0402  [0402]  60.64,91.44 270 top
D20  PESD0402-0402  [0402]  64.33,91.44 270 top
DET  TEST-POINTPOGO_PTH  [1X01_NO_SILK]  39.05,15.24 0 top
DTR  TEST-POINTPOGO_PTH  [1X01_NO_SILK]  101.28,24.13 0 top
ESP32_RF  ANTENNA-SMA-GROUNDEDEDGE_RPSMA  [RP-SMA-EDGE]  75.25,99.31 0 top
ETH_CS  TEST-POINTPOGO_PTH  [1X01_NO_SILK]  100.01,31.75 0 top
ETH_INT  TEST-POINTPOGO_PTH  [1X01_NO_SILK]  97.47,31.75 0 top
F1  6V/2A  [1210]  53.28,50.8 180 top
FB1  600Ω  [0805]  96.58,93.47 0 top
FB2  470Ω  [0603]  45.4,67.31 0 top
FD1  FIDUCIAL1X2  [FIDUCIAL-1X2]  4.76,5.08 0 bottom
FD2  FIDUCIAL1X2  [FIDUCIAL-1X2]  4.76,5.08 0 top
FD3  FIDUCIAL1X2  [FIDUCIAL-1X2]  147,96.52 0 bottom
FD4  FIDUCIAL1X2  [FIDUCIAL-1X2]  147,96.52 0 top
FRAME1  FRAME-LEDGER  [CREATIVE_COMMONS]  not placed on the board
FRAME2  FRAME-LEDGERNO_FOOTPRINT  [DUMMY]  not placed on the board
GND  TEST-POINTPOGO_PTH  [1X01_NO_SILK]  46.67,31.75 90 top
GNSS_RESET  JUMPER-COMBO_2_NO  [COMBO-JUMPER_2_NO]  74.61,77.47 0 bottom
GNSS_RF  ANTENNA-SMA-GROUNDEDEDGE_SMA  [SMA-EDGE]  97.47,99.31 0 top
H1  STAND-OFFTIGHT  [STAND-OFF-TIGHT]  149.54,2.54 0 top
H2  STAND-OFFTIGHT  [STAND-OFF-TIGHT]  149.54,99.06 0 top
H3  STAND-OFFTIGHT  [STAND-OFF-TIGHT]  2.22,99.06 0 top
H4  STAND-OFFTIGHT  [STAND-OFF-TIGHT]  2.22,2.54 0 top
H5  STAND-OFFTIGHT  [STAND-OFF-TIGHT]  65.09,10.16 0 top
H6  STAND-OFFTIGHT  [STAND-OFF-TIGHT]  86.68,10.16 0 top
I2C  JUMPER-SMT_3_NO_SILK  [SMT-JUMPER_3_NO_SILK]  75.88,15.24 0 bottom
I2C1  JUMPER-SMT_3_NO_SILK  [SMT-JUMPER_3_NO_SILK]  110.17,87.63 0 bottom
J1  [USB-C-16P_4LAYER-PADS]  113.98,6.35 0 top
J2  [NANO_SIM_PP]  28.77,7.37 0 top
J3  MICRO-SD-PUSH-PUSH-EXT-PIN  [MICROSD-EXTERNALPIN]  47.94,2.03 0 top
J4  Vertical Qwiic Connector  [JST04_1MM_VERT]  75.88,12.7 180 top
J6  [USB-C-16P_4LAYER-PADS]  139.38,6.35 0 top
J8  [U.FL_REDUCED_FOOTPRINT]  75.25,90.81 90 top
J9  MAGJACK-POE  [MAGJACK-SYM_LED]  14.92,92.2 180 top
J13  [1X10_SCREW_TERMINAL_3.5MM]  46.67,98.42 180 top
L1  2.2uH  [0805-WIDE]  38.04,52.32 270 top
L2  DNP  [0603_NO-CREAM]  136.84,94.23 90 top
L3  DNP  [0603_NO-CREAM]  125.41,94.23 90 top
L4  2.2uH  [0805-WIDE]  42.86,35.56 0 top
LARA_RF1  ANTENNA-SMA-GROUNDEDEDGE_SMA  [SMA-EDGE]  141.92,99.31 0 top
LARA_RF2  ANTENNA-SMA-GROUNDEDEDGE_SMA  [SMA-EDGE]  119.7,99.31 0 top
LED  JUMPER-SMT_2_NC_TRACE_SILK  [SMT-JUMPER_2_NC_TRACE_SILK]  12.38,3.17 0 bottom
LINK  JUMPER-SMT_2_NC_TRACE_SILK  [SMT-JUMPER_2_NC_TRACE_SILK]  20.26,98.42 0 bottom
LOAD  JUMPER-SMT_2_NC_TRACE_SILK  [SMT-JUMPER_2_NC_TRACE_SILK]  42.74,52.07 270 top
LOGO1  SPECIAL_INSTRUCTIONS-ORDERING  [ORDERING_INSTRUCTIONS]  not placed on the board
LOGO2  QWIIC_LOGO_6MM  [QWIIC_6MM]  75.88,15.24 0 top
LOGO4  OSHW-LOGOS  [OSHW-LOGO-S]  124.14,30.48 0 top
LOGO5  SFE_LOGO_NAME.2_INCH  [SFE_LOGO_NAME_.2]  124.14,39.37 0 top
LOGO6  SFE_LOGO_FLAME.2_INCH  [SFE_LOGO_FLAME_.2]  127.7,44.45 0 top
LOGO7  SFE_LOGO_NAME.2_INCH  [SFE_LOGO_NAME_.2]  130.49,71.12 0 bottom
LOGO8  SFE_LOGO_FLAME.2_INCH  [SFE_LOGO_FLAME_.2]  126.94,76.2 0 bottom
MEAS  JUMPER-COMBO_2_NC_TRACE  [COMBO-JUMPER_2_NC_TRACE]  47.94,50.8 0 bottom
NEO_RX  TEST-POINTPOGO_PTH  [1X01_NO_SILK]  73.34,68.58 0 top
NEO_TX  TEST-POINTPOGO_PTH  [1X01_NO_SILK]  73.34,71.12 0 top
PICO  TEST-POINTPOGO_PTH  [1X01_NO_SILK]  47.94,15.24 90 top
PM0  JUMPER-SMT_2_NO_SILK  [SMT-JUMPER_2_NO_SILK]  51.5,82.55 270 bottom
PM1  JUMPER-SMT_2_NO_SILK  [SMT-JUMPER_2_NO_SILK]  53.53,82.55 270 bottom
PM2  JUMPER-SMT_2_NO_SILK  [SMT-JUMPER_2_NO_SILK]  55.56,82.55 270 bottom
POCI  TEST-POINTPOGO_PTH  [1X01_NO_SILK]  41.59,15.24 90 top
PW+  JUMPER-COMBO_2_NC_TRACE  [COMBO-JUMPER_2_NC_TRACE]  9.84,78.74 90 bottom
PW-  JUMPER-COMBO_2_NC_TRACE  [COMBO-JUMPER_2_NC_TRACE]  7.3,78.74 90 bottom
PWREN  TEST-POINTPOGO_PTH  [1X01_NO_SILK]  84.77,25.4 0 top
Q1  [SC70-6]  101.28,20.32 180 top
Q2  [SC70-6]  70.8,43.81 0 top
Q5  310mA/60V/1.6Ω  [SOT323]  129.22,49.53 180 top
Q6  310mA/60V/1.6Ω  [SOT323]  125.41,55.88 180 top
R1  5.1k  [0603]  117.79,11.43 270 top
R2  5.1k  [0603]  110.17,11.43 270 top
R3  10k  [0603]  87.95,30.48 270 top
R4  10k  [0603]  103.82,20.32 90 top
R5  10k  [0603]  98.74,20.32 270 top
R6  33  [0603]  102.55,84.45 90 top
R7  27  [0603]  131.51,30.48 90 top
R8  27  [0603]  133.16,30.48 90 top
R9  27  [0603]  136.46,30.48 90 top
R10  27  [0603]  134.81,30.48 90 top
R11  10k  [0603]  43.5,19.05 90 top
R12  12k  [0603]  138.11,30.48 90 top
R13  1M  [0603]  141.29,24.38 90 top
R14  100k  [0603]  136.72,16.51 90 top
R15  10k  [0603]  82.61,22.86 90 top
R16  2.2k  [0603]  72.07,16.51 90 top
R17  100k  [0603]  130.11,16.51 90 top
R18  100k  [0603]  126.68,24.51 180 top
R19  2.2k  [0603]  79.69,16.51 90 top
R20  100k  [0603]  133.41,16.51 90 top
R21  100k  [0603]  135.06,16.51 270 top
R22  27  [0603]  138.49,16.51 90 top
R23  27  [0603]  140.27,16.51 90 top
R24  1M  [0603]  62.55,78.36 0 top
R25  1k  [0603]  61.91,67.94 180 top
R26  1k  [0603]  61.91,69.85 180 top
R27  33  [0603]  105.85,84.45 90 top
R28  10k  [0603]  104.2,84.45 270 top
R29  12.4k  [0603]  45.4,73.03 0 top
R30  10k  [0603]  51.75,82.55 90 top
R31  10k  [0603]  53.53,82.55 90 top
R32  10k  [0603]  55.31,82.55 90 top
R33  5.1k  [0603]  143.19,11.43 270 top
R34  5.1k  [0603]  135.57,11.43 270 top
R35  49.9  [0603]  35.24,74.93 0 top
R36  33  [0603]  45.4,78.74 180 top
R37  33  [0603]  45.4,80.64 180 top
R38  33  [0603]  45.4,74.93 180 top
R39  33  [0603]  45.4,76.83 180 top
R40  49.9  [0603]  35.24,73.03 0 top
R41  49.9  [0603]  35.24,80.64 180 top
R42  49.9  [0603]  35.24,78.74 180 top
R43  10  [0603]  35.24,82.55 0 top
R44  100k  [0603]  126.81,16.51 90 top
R45  49.9 1/2W  [1206]  42.74,56.01 270 top
R46  33  [0603]  115.76,56.77 270 top
R47  33  [0603]  114.11,56.77 270 top
R48  100k  [0603]  53.02,57.15 0 top
R49  10k  [0603]  58.74,67.31 90 top
R50  100k  [0603]  51.75,38.1 0 top
R51  100k  [0603]  51.75,36.2 0 top
R52  100k  [0603]  128.46,16.51 90 top
R53  1k  [0603]  53.02,54.61 180 top
R54  10k  [0603]  70.8,39.75 0 top
R55  49.9 1/2W  [1206]  59.37,53.59 0 top
R56  1k  [0603]  67.63,45.72 90 top
R57  10k  [0603]  70.8,46.61 180 top
R58  10k  [0603]  53.02,59.69 180 top
R59  49.9 1/2W  [1206]  59.37,50.8 0 top
R60  49.9 1/2W  [1206]  59.37,56.39 0 top
R61  49.9 1/2W  [1206]  59.37,59.18 0 top
R62  470  [0603]  12.38,12.7 180 top
R63  1k  [0603]  67.63,41.91 90 top
R64  10k  [0603]  74.61,75.18 0 top
R65  100k  [0603]  41.85,19.05 90 top
R66  27  [0603]  128.21,30.48 90 top
R67  27  [0603]  129.86,30.48 90 top
R68  1k  [0603]  127.95,55.88 90 top
R69  100k  [0603]  133.41,49.53 270 top
R70  1k  [0603]  131.76,49.53 90 top
R71  2.2k  [0603]  109.41,84.45 90 top
R72  2.2k  [0603]  111.06,84.45 90 top
RESET  MOMENTARY-SWITCH-SPST-PTH-RIGHT-ANGLE-8-020  [TACTILE_SWITCH_PTH_RA_8-020]  101.28,3.81 0 top
RESET_SW  JUMPER-SMT_2_NC_TRACE_SILK  [SMT-JUMPER_2_NC_TRACE_SILK]  101.28,8.89 270 bottom
RTS  TEST-POINTPOGO_PTH  [1X01_NO_SILK]  101.28,16.51 0 top
RX  TEST-POINTPOGO_PTH  [1X01_NO_SILK]  108.9,15.24 0 top
RX2  TEST-POINTPOGO_PTH  [1X01_NO_SILK]  51.75,99.06 0 top
RXD  TEST-POINTPOGO_PTH  [1X01_NO_SILK]  120.33,31.75 0 top
SCK  TEST-POINTPOGO_PTH  [1X01_NO_SILK]  44.13,15.24 90 top
SCL  TEST-POINTPOGO_PTH  [1X01_NO_SILK]  49.21,99.06 0 top
SCL2  TEST-POINTPOGO_PTH  [1X01_NO_SILK]  70.8,11.43 0 top
SD_CS  TEST-POINTPOGO_PTH  [1X01_NO_SILK]  50.48,15.24 90 top
SDA  TEST-POINTPOGO_PTH  [1X01_NO_SILK]  46.67,99.06 0 top
SDA2  TEST-POINTPOGO_PTH  [1X01_NO_SILK]  80.96,11.43 0 top
SHLD1  JUMPER-SMT_2_NC_TRACE_SILK  [SMT-JUMPER_2_NC_TRACE_SILK]  113.98,3.17 270 bottom
SHLD2  JUMPER-SMT_2_NC_TRACE_SILK  [SMT-JUMPER_2_NC_TRACE_SILK]  139.38,3.17 270 bottom
SPWR  JUMPER-SMT_3_1-NC_TRACE_SILK  [SMT-JUMPER_3_1-NC_TRACE_SILK]  56.83,34.29 0 bottom
TP  TEST-POINTPOGO_PTH  [1X01_NO_SILK]  59.37,99.06 0 top
TP_BOOT  TEST-POINTPOGO_PTH  [1X01_NO_SILK]  126.68,12.7 0 top
TP_LED  TEST-POINTPOGO_PTH  [1X01_NO_SILK]  16.19,12.7 0 top
TPWR  JUMPER-SMT_3_1-NC_TRACE_SILK  [SMT-JUMPER_3_1-NC_TRACE_SILK]  61.91,34.29 0 bottom
TX  TEST-POINTPOGO_PTH  [1X01_NO_SILK]  111.44,15.24 0 top
TX2  TEST-POINTPOGO_PTH  [1X01_NO_SILK]  54.29,99.06 0 top
TXD  TEST-POINTPOGO_PTH  [1X01_NO_SILK]  120.33,29.21 0 top
U1  ESP32-WROVER-IE  [ESP32-WROVER-E/IE]  92.39,43.18 180 top
U2  CH340C  [SO016]  112.71,20.32 0 top
U3  XC6222B331MR-G  [SOT23-5]  56.83,30.48 180 top
U4  U-BLOX_ZED-F9P  [ZED-F9P]  108.9,70.48 270 top
U5  U-BLOX_NEO-D9S-00B  [NEO-M9N/M8T/M8U/D9S]  86.04,73.66 0 top
U6  XC6222B331MR-G  [SOT23-5]  51.75,30.48 180 top
U7  W5500  [LQFP-48]  54.29,74.93 270 top
U8  LARA-R6001D  [LARA-LGA]  131.76,72.39 270 top
U9  74LVC4066D_QUAD_BILATERAL_SWITCH  [SO14]  75.88,22.86 0 top
U10  POE_PSU-DP990X  [DP990X]  18.73,63.5 90 top
U11  MCP6021T  [SOT23-5]  63.82,45.72 90 top
U12  AP7361C-33  [UDFN-8]  61.91,30.48 0 top
U13  MCP6021T  [SOT23-5]  63.82,41.91 90 top
U14  BP2G1+_POWER_SPLITTER  [XX21]  96.84,85.09 180 top
U15  USB251XB_USB2514B  [QFN-36]  133.03,24.13 270 top
U16  SN74AVC4T774PW  [SOP65P640X120-16N]  120.33,50.8 270 top
U17  URB2405YMD  [URB_YMD-15WR3]  26.35,36.83 0 top
U18  74HC1G04  [SOT353]  130.49,55.88 180 top
U$2  [33_#_ZED_RXI0]  111.06,45.72 0 bottom
U$3  [#SHLD#0]  140.02,3.17 0 bottom
U$4  [#I�C#0]  110.17,89.34 0 bottom
U$5  [PW#0]  5.4,76.58 90 top
U$6  [PW#1]  11.75,76.58 90 top
U$7  [0_#_BOOT0]  126.81,10.92 0 top
U$8  [#SAFEBOOT#2226]  101.16,87.63 0 bottom
U$9  [#ACT#0]  10.48,98.42 0 bottom
U$10  [#LINK#1]  21.15,98.42 0 bottom
U$11  [RTK_EVK0]  124.14,35.56 0 top
U$12  [#SAFEBOOT#2226]  106.36,92.84 90 top
U$13  [RTK_EVK0]  130.49,67.31 0 bottom
U$14  [NEO_TX2]  77.15,71.12 0 bottom
U$15  [NEO_RX3]  77.15,68.58 0 bottom
U$16  [GND2]  37.91,91.06 90 top
U$17  [3V3_SW20]  61.79,18.67 90 top
U$18  [GND2]  37.91,90.93 270 bottom
U$19  [12_#_SDA20]  80.84,15.88 270 bottom
U$20  [15_#_SCL213]  70.68,15.75 270 bottom
U$21  [ESP32_WIFI_#_BT0]  70.17,101.09 90 top
U$22  [3V3_SW3]  41.47,89.79 90 top
U$23  [3V3_SW3]  41.47,89.66 270 bottom
U$24  [VCCA0]  47.82,66.8 90 top
U$25  [21_#_SDA4]  44.89,89.66 90 top
U$26  [21_#_SDA4]  44.89,89.41 270 bottom
U$28  [22_#_SCL22]  48.32,89.53 90 top
U$29  [27_#_#ETH_CS#0]  105.47,31.88 0 top
U$30  [22_#_SCL22]  48.32,89.41 270 bottom
U$31  [ZED_RX223]  52.01,89.53 90 top
U$32  [ZED_RX223]  52.01,89.41 270 bottom
U$33  [ZED_TX2224]  55.56,89.41 90 top
U$34  [1_#_TX20]  114.87,15.24 0 top
U$35  [3_#_RX20]  105.73,15.24 0 top
U$36  [ZED_TX2224]  55.56,89.15 270 bottom
U$37  [ZED_EXTINT2225]  58.99,88.27 90 top
U$38  [ZED_EXTINT2225]  58.99,88.01 270 bottom
U$39  [ZED_TP2226]  62.55,90.04 90 top
U$40  [ZED_TP2226]  62.55,89.92 270 bottom
U$41  [#SAFEBOOT#2226]  95.06,60.83 90 top
U$42  [ANT_DET2227]  70.8,36.45 0 top
U$43  [#ANT_SHT#2228]  70.68,49.91 0 top
U$44  [9#2230]  46.8,56.13 0 top
U$45  [#SHLD#0]  114.62,3.17 0 bottom
U$46  [#I�C#0]  75.88,16.95 0 bottom
U$47  [99#2230]  49.47,56.13 0 top
U$48  [#I�C#0]  133.03,17.21 0 bottom
U$49  [V_ANT2229]  67.12,58.42 0 top
U$55  [RTS2231]  98.87,16.51 0 top
U$56  [DTR2232]  98.87,24.13 0 top
U$57  [2_#_LED0]  12.26,12.83 0 bottom
U$58  [#LED#2234]  13.27,3.17 0 bottom
U$59  [3V3_SW25]  56.83,23.88 90 top
U$60  [3V325]  51.88,22.61 90 top
U$61  [5V25]  57.72,40.26 0 top
U$62  [MEAS2]  50.61,52.58 0 top
U$63  [VIN#0]  28.51,88.77 270 bottom
U$64  [36_#_SD_DET0]  39.18,9.78 270 bottom
U$65  [3V3_SW20]  61.91,18.54 270 bottom
U$66  [2_#_LED0]  13.53,14.1 0 top
U$67  [#PMODE0#0]  51.5,77.98 270 bottom
U$68  [#PMODE1#1]  53.53,78.11 270 bottom
U$69  [#PMODE2#2]  55.56,77.98 270 bottom
U$70  [VIN#0]  28.51,88.9 90 top
U$71  [VIN#1]  34.35,88.77 270 bottom
U$72  [VIN#1]  34.35,88.9 90 top
U$73  [14_#_RXDO0]  111.32,31.75 0 top
U$74  [#RESET#0]  69.66,77.6 0 bottom
U$75  [13_#_TXDI15]  111.82,29.21 0 top
U$76  [RTS2231]  98.74,16.51 0 bottom
U$77  [DTR2232]  98.74,24.13 0 bottom
U$78  [ESP320]  108.14,3.68 90 top
U$79  [39_#_#ETH_INT#0]  99,30.23 0 top
U$80  [PWR_EN2233]  88.58,25.4 0 bottom
U$81  [V_POE0]  41.85,48.26 0 bottom
U$82  [V_USB3]  41.85,45.72 0 bottom
U$83  [V_USB24]  41.85,43.18 0 bottom
U$84  [MEAS2]  44.89,52.58 0 bottom
U$85  [VIN1]  41.97,40.64 0 bottom
U$86  [5V25]  54.17,40.64 0 bottom
U$87  [3V325]  51.88,18.03 270 bottom
U$88  [3V3_SW25]  56.83,16.64 270 bottom
U$89  [4_#_#SD_CS#15]  50.48,10.92 270 bottom
U$90  [25_#_ZED_TXO0]  111.06,43.18 0 bottom
U$91  [NO0]  86.04,74.93 0 top
U$92  [NO0]  131.76,73.66 0 top
U$93  [#SAFEBOOT#2226]  89.6,66.17 0 bottom
U$94  [ANT_DET2227]  70.55,36.45 0 bottom
U$95  [#ANT_SHT#2228]  66.36,48.39 0 bottom
U$96  [CELLULAR2]  131.76,71.12 0 top
U$97  [L#BAND1]  86.04,72.39 0 top
U$98  [23_#_PICO23]  47.94,10.79 270 bottom
U$99  [1_#_TX20]  114.74,15.24 0 bottom
U$100  [3_#_RX20]  105.6,15.24 0 bottom
U$101  [19_#_POCI19]  41.59,10.92 270 bottom
U$102  [18_#_SCK6]  44.13,11.3 270 bottom
U$103  [13_#_TXDI15]  119.95,31.75 0 bottom
U$104  [99#2230]  49.34,56.13 0 bottom
U$105  [V_ANT2229]  66.99,58.42 0 bottom
U$106  [9#2230]  46.67,56.13 0 bottom
U$107  [VCCA0]  50.99,69.85 0 bottom
U$108  [14_#_RXDO0]  119.95,29.21 0 bottom
U$110  [39_#_#ETH_INT#0]  97.22,31.88 0 bottom
U$111  [27_#_#ETH_CS#0]  105.47,31.88 0 bottom
U$113  [PW#0]  5.4,80.9 270 bottom
U$114  [PW#1]  11.75,81.03 270 bottom
U$115  [VCCIO0]  108.01,54.86 0 top
U$116  [VCCIO0]  111.06,53.34 0 bottom
U$117  [#3V3_SW_EN#0]  55.44,34.29 0 bottom
U$118  [#3V3_SW2_EN#0]  63.31,34.29 0 bottom
U$135  [GND12]  46.67,30.1 0 bottom
U$136  [POE_LOAD0]  31.43,50.8 0 top
U$141  [PWR_EN2233]  88.71,25.4 0 top
U$143  [GND12]  46.67,33.53 0 top
U$146  [HIGH_TEMP_WARNING]  42.86,62.23 0 top
U$147  [HIGH_TEMP_WARNING]  32.19,63.88 0 top
U$148  [RESET0]  101.16,10.92 0 bottom
U$149  [0_#_BOOT0]  126.68,10.92 0 bottom
U$152  [RTK5#SVG0]  139.38,40.13 0 top
U$153  [RTK5#SVG0]  115.25,72.01 0 bottom
U$154  [#GNSS_RESET#0]  81.47,77.6 0 bottom
USB251SCL  [SMT-JUMPER_2_NO_SILK]  134.05,19.05 90 bottom
USB251SDA  [SMT-JUMPER_2_NO_SILK]  132.02,19.05 90 bottom
VANT  TEST-POINTPOGO_PTH  [1X01_NO_SILK]  63.18,58.42 0 top
VCCA  TEST-POINTPOGO_PTH  [1X01_NO_SILK]  47.94,69.85 0 top
VCCIO  TEST-POINTPOGO_PTH  [1X01_NO_SILK]  111.44,53.34 0 top
VID1  10k  [0603]  95.57,30.48 90 top
VID2  1k  [0603]  93.66,30.48 90 top
VIN  TEST-POINTPOGO_PTH  [1X01_NO_SILK]  41.59,40.64 0 top
VIN+  JUMPER-COMBO_2_NC_TRACE  [COMBO-JUMPER_2_NC_TRACE]  30.16,88.9 90 bottom
VIN-  JUMPER-COMBO_2_NC_TRACE  [COMBO-JUMPER_2_NC_TRACE]  32.7,88.9 270 bottom
VPOE  TEST-POINTPOGO_PTH  [1X01_NO_SILK]  41.59,48.26 0 top
VUSB  TEST-POINTPOGO_PTH  [1X01_NO_SILK]  41.59,45.72 0 top
VUSB2  TEST-POINTPOGO_PTH  [1X01_NO_SILK]  41.59,43.18 0 top
Y1  25MHz  [CRYSTAL-SMD-2.0X1.6MM]  62.17,76.07 270 top
Y2  24MHz  [CRYSTAL-SMD-2.0X1.6MM]  139,24.38 0 top
ZED_EXTINT  TEST-POINTPOGO_PTH  [1X01_NO_SILK]  56.83,99.06 0 top
ZED_RXI  TEST-POINTPOGO_PTH  [1X01_NO_SILK]  111.44,45.72 0 top
ZED_TXO  TEST-POINTPOGO_PTH  [1X01_NO_SILK]  111.44,43.18 0 top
